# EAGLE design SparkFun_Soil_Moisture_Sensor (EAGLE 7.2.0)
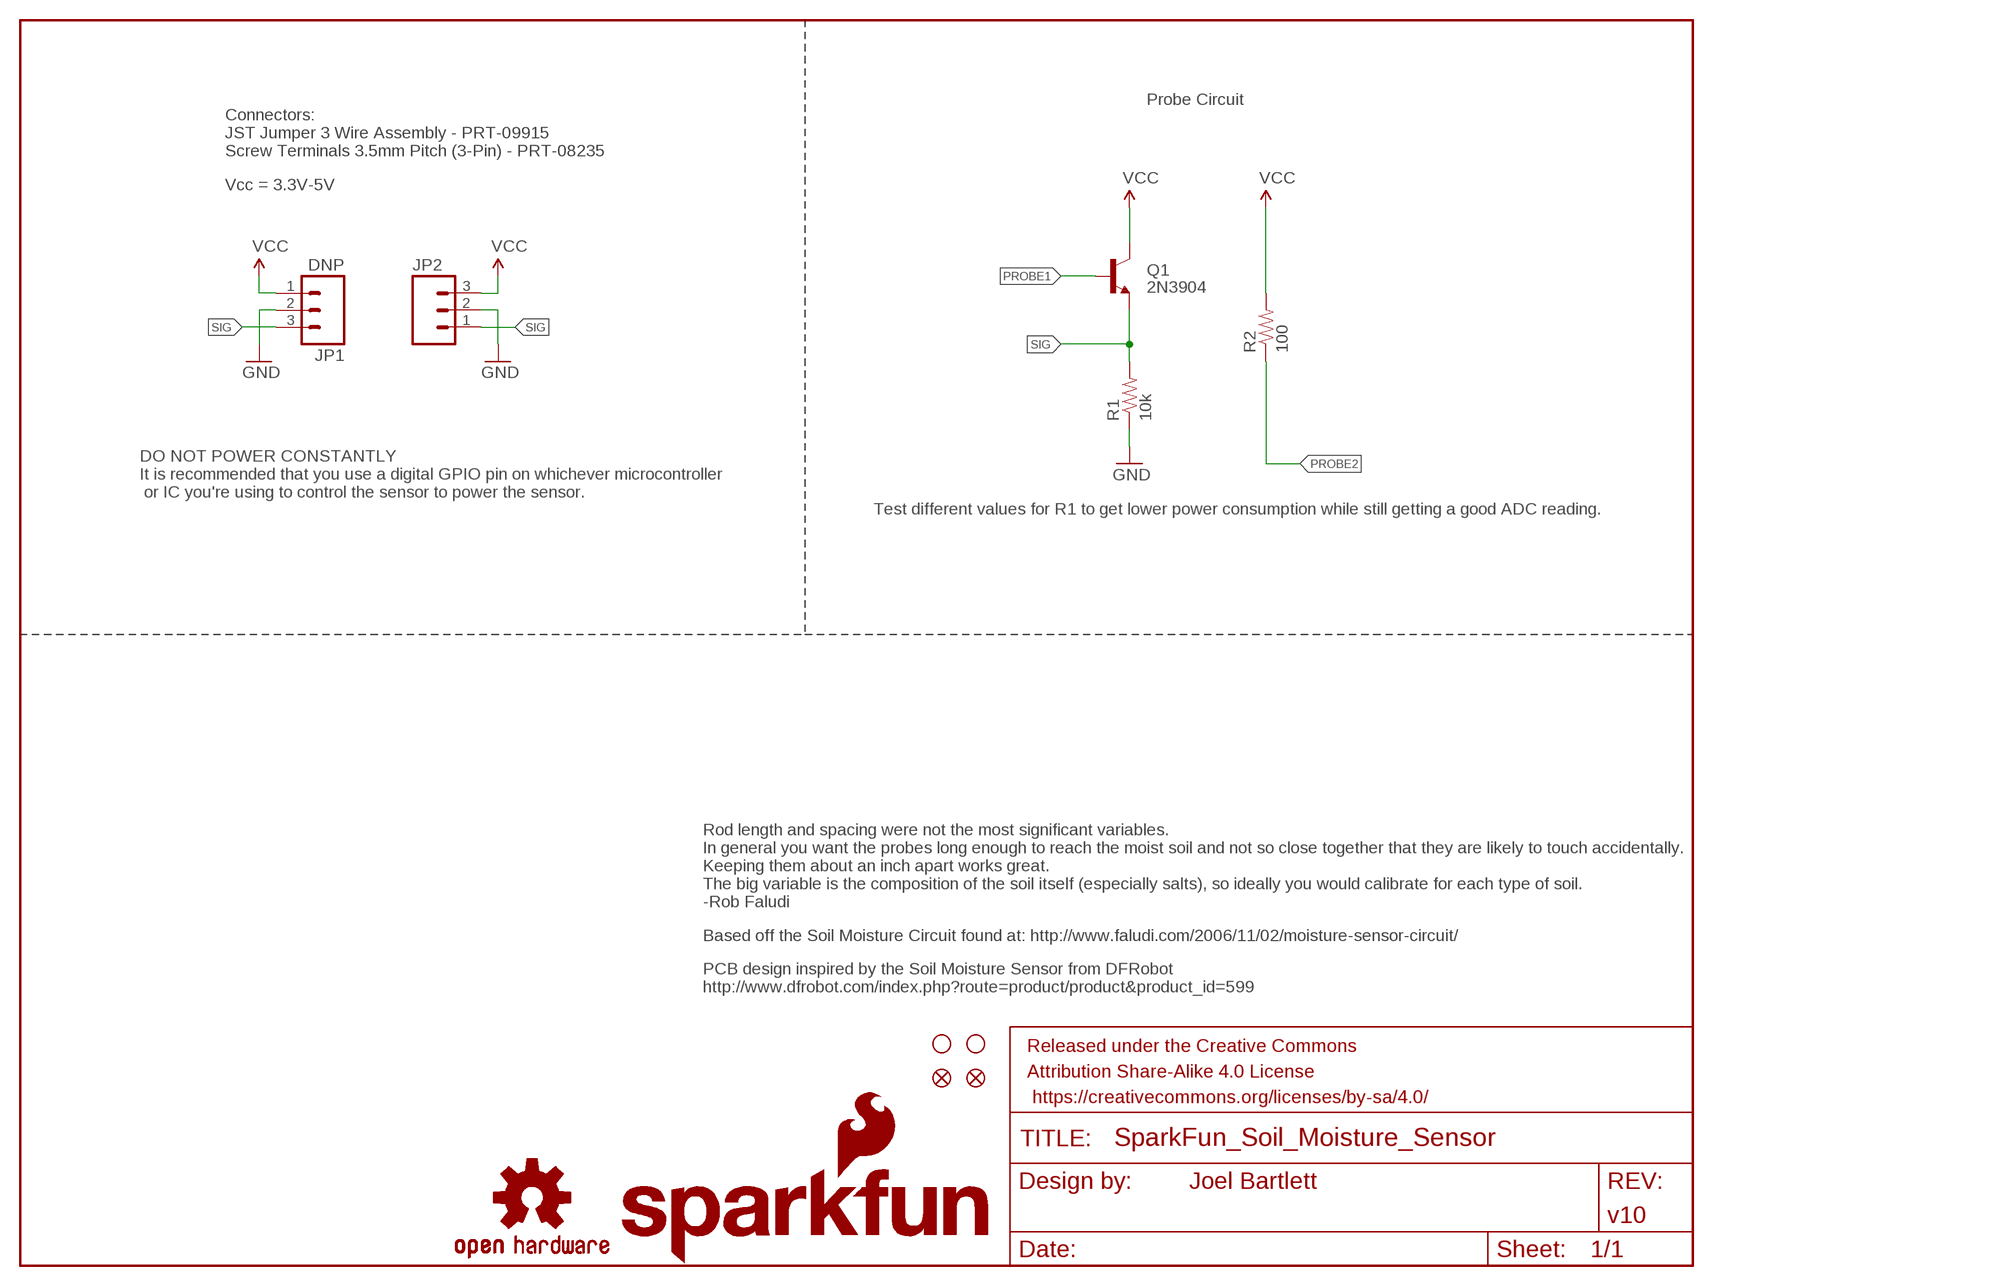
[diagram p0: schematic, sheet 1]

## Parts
FID1  FIDUCIAL1X2  [FIDUCIAL-1X2]
FID2  FIDUCIAL1X2  [FIDUCIAL-1X2]
FRAME1  FRAME-LETTER  [CREATIVE_COMMONS]
JP1  DNP  M03POLAR  [MOLEX-1X3]
JP2  M03SCREW_LOCK  [SCREWTERMINAL-3.5MM-3_LOCK.007S]
LOGO1  SFE_LOGO_NAME_FLAME.1_INCH  [SFE_LOGO_NAME_FLAME_.1]
LOGO2  OSHW-LOGOS  [OSHW-LOGO-S]
Q1  2N3904  TRANSISTOR_NPNMMBT2222A  [SOT23-3]
R1  10k  100OHM-1/4W-5%(0603)  [0603-RES]
R2  100  100OHM-1/4W-5%(0603)  [0603-RES]
STANDOFF1  STAND-OFF  [STAND-OFF]
STANDOFF2  STAND-OFF  [STAND-OFF]

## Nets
GND: JP1.2 JP2.2 R1.1
PROBE1: Q1.1(B)
PROBE2: R2.1
SIG: JP1.3 JP2.1 Q1.2(E) R1.2
VCC: JP1.1 JP2.3 Q1.3(C) R2.2

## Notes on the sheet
- Probe Circuit
- Connectors: 
  JST Jumper 3 Wire Assembly - PRT-09915
  Screw Terminals 3.5mm Pitch (3-Pin) - PRT-08235
- Vcc = 3.3V-5V
- DO NOT POWER CONSTANTLY 
  It is recommended that you use a digital GPIO pin on whichever microcontroller
   or IC you're using to control the sensor to power the sensor.
- Test different values for R1 to get lower power consumption while still getting a good ADC reading.
- Rod length and spacing were not the most significant variables. 
  In general you want the probes long enough to reach the moist soil and not so close together that they are likely to touch accidentally. 
  Keeping them about an inch apart works great. 
  The big variable is the composition of the soil itself (especially salts), so ideally you would calibrate for each type of soil. 
  -Rob Faludi
- Based off the Soil Moisture Circuit found at: http://www.faludi.com/2006/11/02/moisture-sensor-circuit/
- PCB design inspired by the Soil Moisture Sensor from DFRobot
  http://www.dfrobot.com/index.php?route=product/product&product_id=599

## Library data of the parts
FID1 FID2 = SparkFun-Aesthetics:FIDUCIAL: Fiducial Alignment Points
FRAME1 = SparkFun-Aesthetics:FRAME-LETTER: Schematic Frame; DESIGNER: Joel Bartlett; VERSION: v10
JP1 = SparkFun-Connectors:M03: Header 3 Standard 3-pin 0.1" header. Use with straight break away headers (SKU : PRT-00116), right angle break away headers (PRT-00553), swiss pins (PRT-00743), machine pins (PRT-00117), and female headers (PRT-00115). Molex polarized connector foot print use with SKU : PRT-08232 with associated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
JP2 = SparkFun-Connectors:M03: Header 3 Standard 3-pin 0.1" header. Use with straight break away headers (SKU : PRT-00116), right angle break away headers (PRT-00553), swiss pins (PRT-00743), machine pins (PRT-00117), and female headers (PRT-00115). Molex polarized connector foot print use with SKU : PRT-08232 with associated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; PROD_ID: CONN-08288
LOGO1 = SparkFun-Aesthetics:SFE_LOGO_NAME_FLAME: SFE Logo, name and flame
LOGO2 = SparkFun-Aesthetics:OSHW-LOGO: Open Source Hardware Logo
Q1 = SparkFun-DiscreteSemi:TRANSISTOR_NPN: Generic NPN BJT MMBT2222A - TRANS-08049 (SOT-23, 1A 40V) MPSA42 - TRANS-09116 (SOT-23, 500mA 300V) MMBT5088LT1G - TRANS-11160 (SOT-23, 50 mA 30V) BC547 - COM-08928 (TO-92 45V 100mA) (1.Collector 2.Base 3.Emitter) 2N3904 - COM-00521 (TO-92 40V 200mA) (1.Emitter 2.Base 3.Collector) P2N2222A -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; PROD_ID: TRANS-08049; VALUE: MMBT2222A
R1 R2 = SparkFun-Resistors:100OHM-1/4W-5%(0603); PROD_ID: RES-12438; VALUE: 100/.25W
STANDOFF1 STANDOFF2 = SparkFun-Electromechanical:STAND-OFF: #4 Stand Off

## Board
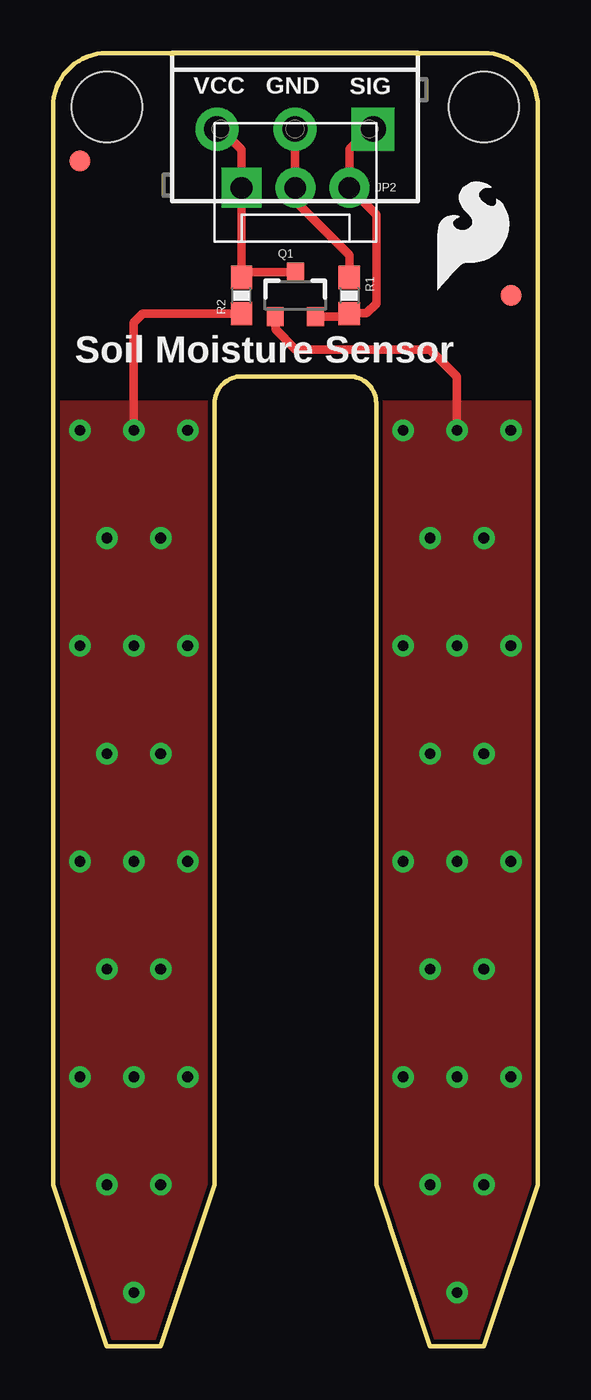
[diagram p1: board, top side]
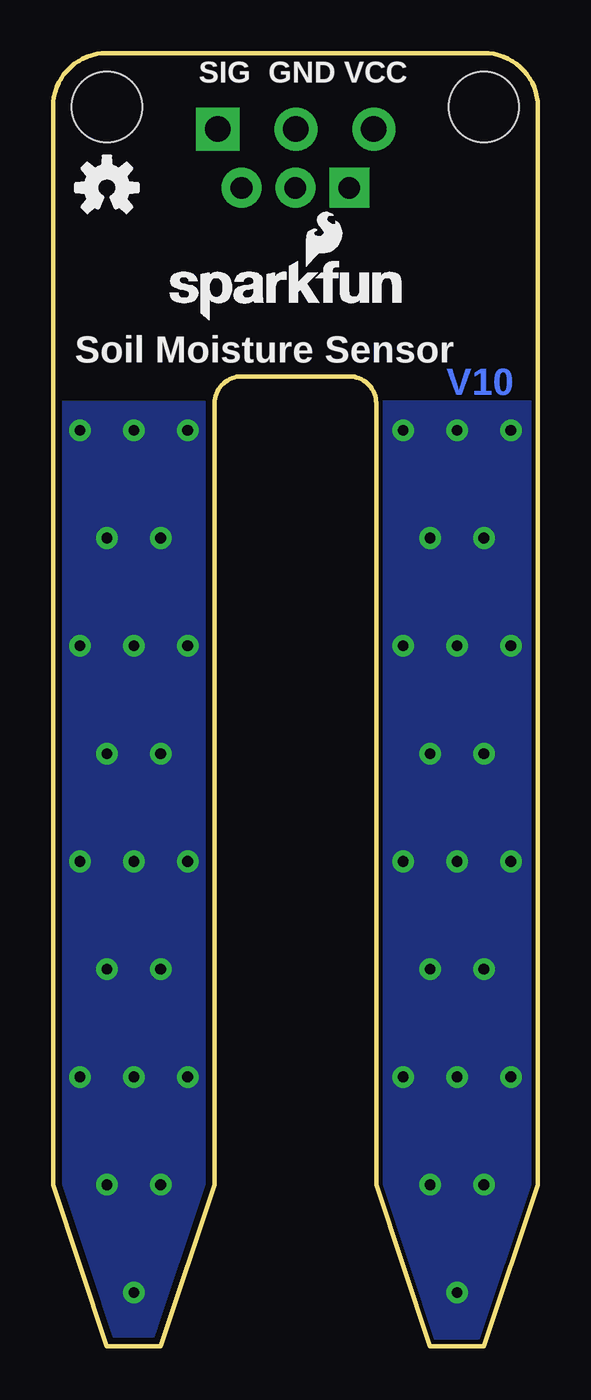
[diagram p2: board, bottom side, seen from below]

Size 22.86 x 60.96 mm. Coordinates in mm from the lower left corner, seen from the top.
Outline: 2.54,60.96 arc90 0,58.42 0,7.62 2.54,0 5.08,0 7.62,7.62 7.62,44.45 arc-90 8.89,45.72 13.97,45.72 arc-90 15.24,44.45 15.24,7.62 17.78,0 20.32,0 22.86,7.62 22.86,58.42 arc90 20.32,60.96 2.54,60.96
Copper layers (1*16): Top 0.035mm / dielectric 1.5mm / Bottom 0.035mm
Design rules "SparkFun-2-layer": minimum track width 7mil, minimum drill 15mil, track to track 8mil, track to pad 8mil, pad to pad 8mil, via to via 8mil, smd to smd 8mil, copper to edge 8mil, drill to drill 8mil, minimum pad ring 12mil, minimum via ring 10mil, stop-mask expansion 4mil, vias tented up to drill 20mil, thermal gap 10mil

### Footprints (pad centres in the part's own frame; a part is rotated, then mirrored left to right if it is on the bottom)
FIDUCIAL-1X2 = smd 1 x 1: 1 0,0
MOLEX-1X3 = drill 1.016 pad 1.88 square: 1 0,0 | drill 1.016 pad 1.88: 2 2.54,0; 3 5.08,0
SCREWTERMINAL-3.5MM-3_LOCK.007S = drill 1.2 pad 2.032 square: 1 -0.178,0 | drill 1.2 pad 2.032: 2 3.5,0; 3 7.178,0
SOT23-3 = smd 0.8 x 0.9: 1 -0.95,-1; 2 0.95,-1; 3 0,1.1
0603-RES = smd 1.1 x 1: 1 -0.85,0; 2 0.85,0
STAND-OFF = hole 3.302: 0,0

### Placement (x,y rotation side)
FID1  1.27,55.88 0 top
FID2  21.59,49.53 0 top
FRAME1  not placed on the board
JP1  8.89,54.61 0 top
JP2  14.91,57.38 180 top
LOGO1  17.78,48.26 0 bottom
LOGO2  20.32,54.61 0 bottom
Q1  11.43,49.53 0 top
R1  13.97,49.53 270 top
R2  8.89,49.53 90 top
STANDOFF1  2.54,58.42 0 top
STANDOFF2  20.32,58.42 0 top
U$4  [SFE_LOGO_FLAME_.2]  17.78,49.53 0 top

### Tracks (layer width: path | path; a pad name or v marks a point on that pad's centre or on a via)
GND
  Top 0.254: 11.41,54.63 JP1.2
  Top 0.406: JP1.2 11.43,53.98 13.97,51.44 R1.1 | 11.41,54.63 JP2.2
PROBE1  (via drill 0.51)
  Top 0.406: Q1.1 10.48,47.94 11.43,46.99 17.78,46.99 19.05,45.72 v19.05,43.18
  other vias: 16.51,43.18 21.59,43.18 21.59,33.02 19.05,33.02 16.51,33.02 16.51,22.86 19.05,22.86 21.59,22.86 21.59,12.7 19.05,12.7 16.51,12.7 17.78,7.62 20.32,7.62 19.05,2.54 17.78,38.1 20.32,38.1 20.32,27.94 17.78,27.94 17.78,17.78 20.32,17.78
  pour Top: 15.24,44.45 15.24,0 22.86,0 22.86,44.45
  pour Bottom (isolate 0.305): 15.24,44.45 15.24,0 22.86,0 22.86,44.45
PROBE2  (via drill 0.51)
  Top 0.406: v3.81,43.18 3.81,48.26 4.23,48.68 R2.1
  other vias: 6.35,43.18 1.27,43.18 1.27,33.02 3.81,33.02 6.35,33.02 6.35,22.86 3.81,22.86 1.27,22.86 1.27,12.7 3.81,12.7 6.35,12.7 5.08,7.62 2.54,7.62 3.81,2.54 2.54,17.78 5.08,17.78 2.54,27.94 5.08,27.94 2.54,38.1 5.08,38.1
  pour Top: 0,44.45 0,0 7.62,0 7.62,44.45
  pour Bottom: 0,44.45 0,0 7.62,0 7.62,44.45
SIG
  Top 0.254: 13.82,48.53 R1.2 13.98,48.69
  Top 0.406: Q1.2 13.82,48.53 | 13.98,48.69 14.78,48.69 15.24,49.15 15.24,53.34 JP1.3 13.97,56.44 14.91,57.38 JP2.1
VCC
  Top 0.254: R2.2 9.14,50.63
  Top 0.406: 9.14,50.63 Q1.3 | R2.2 JP1.1 8.89,56.4 7.91,57.38 JP2.3

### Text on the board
Bottom: V10
tPlace: VCC | GND | SIG | Soil Moisture Sensor
bPlace: VCC | GND | SIG | Soil Moisture Sensor
tDocu: Joel Bartlett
